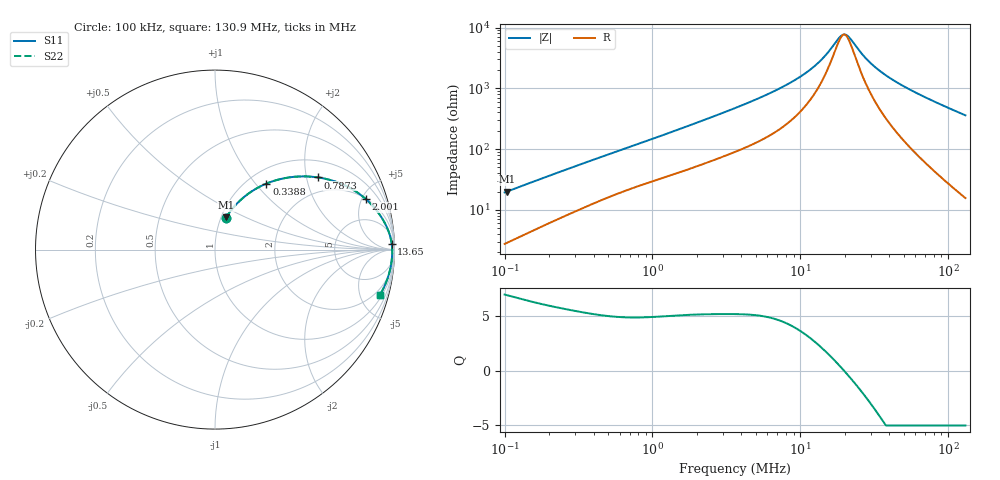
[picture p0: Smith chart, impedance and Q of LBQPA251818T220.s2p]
! LBQPA251818T220  S-PARAMETER MODEL  ( General Type )
! Model Generated by TAIYO YUDEN Corporation (http://www.ty-top.com)
! Version 1.0
! TAIYO YUDEN Control No. 191025NI43SB-FBB
! Copyright(c) 2019 TAIYO YUDEN CO.,LTD. All Rights Reserved.
! Product Description (link to TY-COMPAS)
! https://ds.yuden.co.jp/TYCOMPAS/or/detail?pn=LBQPA251818T220K&u=M
! Products Name : Inductors
! Characteristics :
!  Inductance : 22 uH , SRF(min) : 19 MHz , DC Resistance(max) : 1.001 Ohm
!  Rated Current : Saturation :320 mA , Temp Rise : 250 mA (20 degC)
!  Case Size : 2.5 x 1.8 / 0.098 x 0.071 [mm/inch] , Thickness : 1.8 / 0.071 [mm/inch]
!  (Conditions: Temperature = 25 degC , DC Bias Current/Voltage = 0A / 0V)
! External Node Assignments :
!  1  o---GGG---o  2
! GND o---------o GND
! Frequency Range : 0.1MHz  -  130.914307MHz  [ 402 STEP ]
# MHz S RI R 50
! Freq[MHz].  S11 Real  S11 Imag  S21 Real  S21 Imag  S12 Real  S12 Imag  S22 Real  S22 Imag
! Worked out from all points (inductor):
!   401 points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, 100 kHz to 130.9 MHz, reference 50 ohm
!   read as one part in series: L = 29.8 uH near 103.7 kHz
!   highest Q = 6.89 at 103.7 kHz (marker M1), where L = 30.4 uH
!   self-resonance near 19.78 MHz
!   S11 on the Smith chart (normalised r, x): 100 kHz: 1.06, +0.38; 338.8 kHz: 1.21, +1.14; 787.3 kHz: 1.48, +2.35; 2.001 MHz: 2.04, +5.35; 13.65 MHz: 24, +51; 130.9 MHz: 1.31, -7.18
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0.1  0.0594 0.1752  0.9406 -0.1752  0.9406 -0.1752  0.0594 0.1752
0.103654  0.0626 0.1803  0.9374 -0.1803  0.9374 -0.1803  0.0626 0.1803
0.190778  0.1447 0.2781  0.8553 -0.2781  0.8553 -0.2781  0.1447 0.2781
0.332733  0.2808 0.3654  0.7192 -0.3654  0.7192 -0.3654  0.2808 0.3654
0.338757  0.2862 0.3677  0.7138 -0.3677  0.7138 -0.3677  0.2862 0.3677
0.521083  0.429 0.4043  0.571 -0.4043  0.571 -0.4043  0.429 0.4043
0.787288  0.5747 0.402  0.4253 -0.402  0.4253 -0.402  0.5747 0.402
1.10711  0.6878 0.373  0.3122 -0.373  0.3122 -0.373  0.6878 0.373
2.001438  0.8392 0.2825  0.1608 -0.2825  0.1608 -0.2825  0.8392 0.2825
3.683715  0.9262 0.182  0.0738 -0.182  0.0738 -0.182  0.9262 0.182
7.416385  0.9709 0.0908  0.0291 -0.0908  0.0291 -0.0908  0.9709 0.0908
9.706872  0.9789 0.0627  0.0211 -0.0627  0.0211 -0.0627  0.9789 0.0627
12.03896  0.9829 0.0424  0.0171 -0.0424  0.0171 -0.0424  0.9829 0.0424
13.65011  0.9846 0.0313  0.0154 -0.0313  0.0154 -0.0313  0.9846 0.0313
18.5186  0.9869 0.00547  0.0131 -0.00547  0.0131 -0.00547  0.9869 0.00547
20.25678  0.9872 -0.002  0.0128 0.002  0.0128 0.002  0.9872 -0.002
21.76408  0.9873 -0.00801  0.0127 0.00801  0.0127 0.00801  0.9873 -0.00801
26.04144  0.9872 -0.0233  0.0128 0.0233  0.0128 0.0233  0.9872 -0.0233
29.52652  0.9867 -0.0344  0.0133 0.0344  0.0133 0.0344  0.9867 -0.0344
40.05754  0.9841 -0.064  0.0159 0.064  0.0159 0.064  0.9841 -0.064
66.20234  0.9721 -0.1259  0.0279 0.1259  0.0279 0.1259  0.9721 -0.1259
130.9143  0.9187 -0.2524  0.0813 0.2524  0.0813 0.2524  0.9187 -0.2524
